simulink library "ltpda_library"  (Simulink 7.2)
settings: Solver=ode45  SolverMode=SingleTasking  StartTime=0.0  StopTime=10.0  RelTol=1e-3
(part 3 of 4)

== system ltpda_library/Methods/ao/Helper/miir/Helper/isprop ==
  In1 : Inport  OutDataType=sfix(16)  OutScaling=2^0
  isprop : M-S-Function  Tag=isprop  FunctionName=ltpdasim
  Out1 : Outport  OutDataType=sfix(16)  OutScaling=2^0
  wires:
  In1/1 -> isprop/1
  isprop/1 -> Out1/1

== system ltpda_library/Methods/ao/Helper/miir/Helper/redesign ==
  In1 : Inport  OutDataType=sfix(16)  OutScaling=2^0
  redesign : M-S-Function  Tag=redesign  FunctionName=ltpdasim
  Out1 : Outport  OutDataType=sfix(16)  OutScaling=2^0
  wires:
  In1/1 -> redesign/1
  redesign/1 -> Out1/1

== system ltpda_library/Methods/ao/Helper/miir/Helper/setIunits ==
  In1 : Inport  OutDataType=sfix(16)  OutScaling=2^0
  setIunits : M-S-Function  Tag=setIunits  FunctionName=ltpdasim
  Out1 : Outport  OutDataType=sfix(16)  OutScaling=2^0
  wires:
  In1/1 -> setIunits/1
  setIunits/1 -> Out1/1

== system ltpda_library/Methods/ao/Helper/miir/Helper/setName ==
  In1 : Inport  OutDataType=sfix(16)  OutScaling=2^0
  setName : M-S-Function  Tag=setName  FunctionName=ltpdasim
  Out1 : Outport  OutDataType=sfix(16)  OutScaling=2^0
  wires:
  In1/1 -> setName/1
  setName/1 -> Out1/1

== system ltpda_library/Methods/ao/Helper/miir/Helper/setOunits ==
  In1 : Inport  OutDataType=sfix(16)  OutScaling=2^0
  setOunits : M-S-Function  Tag=setOunits  FunctionName=ltpdasim
  Out1 : Outport  OutDataType=sfix(16)  OutScaling=2^0
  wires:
  In1/1 -> setOunits/1
  setOunits/1 -> Out1/1

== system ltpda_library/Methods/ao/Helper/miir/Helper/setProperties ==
  In1 : Inport  OutDataType=sfix(16)  OutScaling=2^0
  setProperties : M-S-Function  Tag=setProperties  FunctionName=ltpdasim
  Out1 : Outport  OutDataType=sfix(16)  OutScaling=2^0
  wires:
  In1/1 -> setProperties/1
  setProperties/1 -> Out1/1

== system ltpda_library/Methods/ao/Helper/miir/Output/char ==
  In1 : Inport  OutDataType=sfix(16)  OutScaling=2^0
  Terminator : Terminator
  char : M-S-Function  Tag=char  FunctionName=ltpdasim
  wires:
  char/1 -> Terminator/1
  In1/1 -> char/1

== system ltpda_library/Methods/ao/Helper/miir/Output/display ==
  In1 : Inport  OutDataType=sfix(16)  OutScaling=2^0
  Terminator : Terminator
  display : M-S-Function  Tag=display  FunctionName=ltpdasim
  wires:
  display/1 -> Terminator/1
  In1/1 -> display/1

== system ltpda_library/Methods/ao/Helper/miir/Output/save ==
  In1 : Inport  OutDataType=sfix(16)  OutScaling=2^0
  Terminator : Terminator
  report : M-S-Function  Tag=report  FunctionName=ltpdasim
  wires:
  report/1 -> Terminator/1
  In1/1 -> report/1

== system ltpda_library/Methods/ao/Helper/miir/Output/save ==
  In1 : Inport  OutDataType=sfix(16)  OutScaling=2^0
  Terminator : Terminator
  save : M-S-Function  Tag=save  FunctionName=ltpdasim
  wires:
  save/1 -> Terminator/1
  In1/1 -> save/1

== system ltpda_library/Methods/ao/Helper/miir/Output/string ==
  In1 : Inport  OutDataType=sfix(16)  OutScaling=2^0
  Terminator : Terminator
  string : M-S-Function  Tag=string  FunctionName=ltpdasim
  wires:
  string/1 -> Terminator/1
  In1/1 -> string/1

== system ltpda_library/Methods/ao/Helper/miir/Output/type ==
  In1 : Inport  OutDataType=sfix(16)  OutScaling=2^0
  Terminator : Terminator
  type : M-S-Function  Tag=type  FunctionName=ltpdasim
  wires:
  type/1 -> Terminator/1
  In1/1 -> type/1

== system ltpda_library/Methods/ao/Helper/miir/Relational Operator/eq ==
  In1 : Inport  OutDataType=sfix(16)  OutScaling=2^0
  eq : M-S-Function  Tag=eq  FunctionName=ltpdasim
  Out1 : Outport  OutDataType=sfix(16)  OutScaling=2^0
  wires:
  In1/1 -> eq/1
  eq/1 -> Out1/1

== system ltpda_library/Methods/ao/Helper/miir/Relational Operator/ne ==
  In1 : Inport  OutDataType=sfix(16)  OutScaling=2^0
  ne : M-S-Function  Tag=ne  FunctionName=ltpdasim
  Out1 : Outport  OutDataType=sfix(16)  OutScaling=2^0
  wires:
  In1/1 -> ne/1
  ne/1 -> Out1/1

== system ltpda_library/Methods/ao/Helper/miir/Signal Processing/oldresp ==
  In1 : Inport  OutDataType=sfix(16)  OutScaling=2^0
  oldresp : M-S-Function  Tag=oldresp  FunctionName=ltpdasim
  Out1 : Outport  OutDataType=sfix(16)  OutScaling=2^0
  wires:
  In1/1 -> oldresp/1
  oldresp/1 -> Out1/1

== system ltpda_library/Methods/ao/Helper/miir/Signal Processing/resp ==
  In1 : Inport  OutDataType=sfix(16)  OutScaling=2^0
  resp : M-S-Function  Tag=resp  FunctionName=ltpdasim
  Out1 : Outport  OutDataType=sfix(16)  OutScaling=2^0
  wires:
  In1/1 -> resp/1
  resp/1 -> Out1/1

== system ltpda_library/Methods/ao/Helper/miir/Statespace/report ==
  In1 : Inport  OutDataType=sfix(16)  OutScaling=2^0
  report : M-S-Function  Tag=report  FunctionName=ltpdasim
  Out1 : Outport  OutDataType=sfix(16)  OutScaling=2^0
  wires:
  In1/1 -> report/1
  report/1 -> Out1/1

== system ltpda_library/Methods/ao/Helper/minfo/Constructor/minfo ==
  Ground : Ground
  minfo : M-S-Function  Tag=minfo  FunctionName=ltpdasim
  Out1 : Outport  OutDataType=sfix(16)  OutScaling=2^0
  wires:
  Ground/1 -> minfo/1
  minfo/1 -> Out1/1

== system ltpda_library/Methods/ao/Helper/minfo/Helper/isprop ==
  In1 : Inport  OutDataType=sfix(16)  OutScaling=2^0
  isprop : M-S-Function  Tag=isprop  FunctionName=ltpdasim
  Out1 : Outport  OutDataType=sfix(16)  OutScaling=2^0
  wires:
  In1/1 -> isprop/1
  isprop/1 -> Out1/1

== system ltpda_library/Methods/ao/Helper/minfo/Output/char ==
  In1 : Inport  OutDataType=sfix(16)  OutScaling=2^0
  Terminator : Terminator
  char : M-S-Function  Tag=char  FunctionName=ltpdasim
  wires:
  char/1 -> Terminator/1
  In1/1 -> char/1

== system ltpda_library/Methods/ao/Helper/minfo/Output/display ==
  In1 : Inport  OutDataType=sfix(16)  OutScaling=2^0
  Terminator : Terminator
  display : M-S-Function  Tag=display  FunctionName=ltpdasim
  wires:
  display/1 -> Terminator/1
  In1/1 -> display/1

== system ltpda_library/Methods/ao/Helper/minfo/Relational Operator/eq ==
  In1 : Inport  OutDataType=sfix(16)  OutScaling=2^0
  eq : M-S-Function  Tag=eq  FunctionName=ltpdasim
  Out1 : Outport  OutDataType=sfix(16)  OutScaling=2^0
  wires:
  In1/1 -> eq/1
  eq/1 -> Out1/1

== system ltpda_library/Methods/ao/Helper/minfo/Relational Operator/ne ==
  In1 : Inport  OutDataType=sfix(16)  OutScaling=2^0
  ne : M-S-Function  Tag=ne  FunctionName=ltpdasim
  Out1 : Outport  OutDataType=sfix(16)  OutScaling=2^0
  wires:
  In1/1 -> ne/1
  ne/1 -> Out1/1

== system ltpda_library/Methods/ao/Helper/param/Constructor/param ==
  Ground : Ground
  param : M-S-Function  Tag=param  FunctionName=ltpdasim
  Out1 : Outport  OutDataType=sfix(16)  OutScaling=2^0
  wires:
  Ground/1 -> param/1
  param/1 -> Out1/1

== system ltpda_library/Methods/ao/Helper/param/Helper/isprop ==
  In1 : Inport  OutDataType=sfix(16)  OutScaling=2^0
  isprop : M-S-Function  Tag=isprop  FunctionName=ltpdasim
  Out1 : Outport  OutDataType=sfix(16)  OutScaling=2^0
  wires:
  In1/1 -> isprop/1
  isprop/1 -> Out1/1

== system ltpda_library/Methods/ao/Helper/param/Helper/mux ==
  In1 : Inport  OutDataType=sfix(16)  OutScaling=2^0
  mux : M-S-Function  Tag=mux  FunctionName=ltpdasim
  Out1 : Outport  OutDataType=sfix(16)  OutScaling=2^0
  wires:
  In1/1 -> mux/1
  mux/1 -> Out1/1

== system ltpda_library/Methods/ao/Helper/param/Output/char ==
  In1 : Inport  OutDataType=sfix(16)  OutScaling=2^0
  Terminator : Terminator
  char : M-S-Function  Tag=char  FunctionName=ltpdasim
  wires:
  char/1 -> Terminator/1
  In1/1 -> char/1

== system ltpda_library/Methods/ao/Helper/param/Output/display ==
  In1 : Inport  OutDataType=sfix(16)  OutScaling=2^0
  Terminator : Terminator
  display : M-S-Function  Tag=display  FunctionName=ltpdasim
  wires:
  display/1 -> Terminator/1
  In1/1 -> display/1

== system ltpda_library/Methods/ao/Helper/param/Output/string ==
  In1 : Inport  OutDataType=sfix(16)  OutScaling=2^0
  Terminator : Terminator
  string : M-S-Function  Tag=string  FunctionName=ltpdasim
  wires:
  string/1 -> Terminator/1
  In1/1 -> string/1

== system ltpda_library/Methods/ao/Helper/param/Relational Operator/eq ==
  In1 : Inport  OutDataType=sfix(16)  OutScaling=2^0
  eq : M-S-Function  Tag=eq  FunctionName=ltpdasim
  Out1 : Outport  OutDataType=sfix(16)  OutScaling=2^0
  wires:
  In1/1 -> eq/1
  eq/1 -> Out1/1

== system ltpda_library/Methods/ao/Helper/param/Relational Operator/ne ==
  In1 : Inport  OutDataType=sfix(16)  OutScaling=2^0
  ne : M-S-Function  Tag=ne  FunctionName=ltpdasim
  Out1 : Outport  OutDataType=sfix(16)  OutScaling=2^0
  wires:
  In1/1 -> ne/1
  ne/1 -> Out1/1

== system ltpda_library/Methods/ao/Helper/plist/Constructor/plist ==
  Ground : Ground
  plist : M-S-Function  Tag=plist  FunctionName=ltpdasim
  Out1 : Outport  OutDataType=sfix(16)  OutScaling=2^0
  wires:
  Ground/1 -> plist/1
  ?parfrac/1 -> Out1/1

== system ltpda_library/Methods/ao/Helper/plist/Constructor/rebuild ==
  Ground : Ground
  rebuild : M-S-Function  Tag=rebuild  FunctionName=ltpdasim
  Out1 : Outport  OutDataType=sfix(16)  OutScaling=2^0
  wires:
  Ground/1 -> rebuild/1
  rebuild/1 -> Out1/1

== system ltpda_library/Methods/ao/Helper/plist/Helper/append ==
  In1 : Inport  OutDataType=sfix(16)  OutScaling=2^0
  append : M-S-Function  Tag=append  FunctionName=ltpdasim
  Out1 : Outport  OutDataType=sfix(16)  OutScaling=2^0
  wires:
  In1/1 -> append/1
  append/1 -> Out1/1

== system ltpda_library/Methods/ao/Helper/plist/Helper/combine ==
  In1 : Inport  OutDataType=sfix(16)  OutScaling=2^0
  combine : M-S-Function  Tag=combine  FunctionName=ltpdasim
  Out1 : Outport  OutDataType=sfix(16)  OutScaling=2^0
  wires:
  In1/1 -> combine/1
  combine/1 -> Out1/1

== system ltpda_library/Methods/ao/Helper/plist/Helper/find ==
  In1 : Inport  OutDataType=sfix(16)  OutScaling=2^0
  find : M-S-Function  Tag=find  FunctionName=ltpdasim
  Out1 : Outport  OutDataType=sfix(16)  OutScaling=2^0
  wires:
  In1/1 -> find/1
  find/1 -> Out1/1

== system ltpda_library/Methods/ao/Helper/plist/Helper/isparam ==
  In1 : Inport  OutDataType=sfix(16)  OutScaling=2^0
  isparam : M-S-Function  Tag=isparam  FunctionName=ltpdasim
  Out1 : Outport  OutDataType=sfix(16)  OutScaling=2^0
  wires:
  In1/1 -> isparam/1
  isparam/1 -> Out1/1

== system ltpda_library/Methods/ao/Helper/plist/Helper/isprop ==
  In1 : Inport  OutDataType=sfix(16)  OutScaling=2^0
  isprop : M-S-Function  Tag=isprop  FunctionName=ltpdasim
  Out1 : Outport  OutDataType=sfix(16)  OutScaling=2^0
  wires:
  In1/1 -> isprop/1
  isprop/1 -> Out1/1

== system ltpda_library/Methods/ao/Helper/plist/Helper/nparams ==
  In1 : Inport  OutDataType=sfix(16)  OutScaling=2^0
  nparams : M-S-Function  Tag=nparams  FunctionName=ltpdasim
  Out1 : Outport  OutDataType=sfix(16)  OutScaling=2^0
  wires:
  In1/1 -> nparams/1
  nparams/1 -> Out1/1

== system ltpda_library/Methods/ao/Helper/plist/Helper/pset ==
  In1 : Inport  OutDataType=sfix(16)  OutScaling=2^0
  pset : M-S-Function  Tag=pset  FunctionName=ltpdasim
  Out1 : Outport  OutDataType=sfix(16)  OutScaling=2^0
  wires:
  In1/1 -> pset/1
  pset/1 -> Out1/1

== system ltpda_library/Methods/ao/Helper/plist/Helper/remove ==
  In1 : Inport  OutDataType=sfix(16)  OutScaling=2^0
  remove : M-S-Function  Tag=remove  FunctionName=ltpdasim
  Out1 : Outport  OutDataType=sfix(16)  OutScaling=2^0
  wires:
  In1/1 -> remove/1
  remove/1 -> Out1/1

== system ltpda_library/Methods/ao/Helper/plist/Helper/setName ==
  In1 : Inport  OutDataType=sfix(16)  OutScaling=2^0
  setName : M-S-Function  Tag=setName  FunctionName=ltpdasim
  Out1 : Outport  OutDataType=sfix(16)  OutScaling=2^0
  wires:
  In1/1 -> setName/1
  setName/1 -> Out1/1

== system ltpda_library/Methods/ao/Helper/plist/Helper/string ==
  In1 : Inport  OutDataType=sfix(16)  OutScaling=2^0
  string : M-S-Function  Tag=string  FunctionName=ltpdasim
  Out1 : Outport  OutDataType=sfix(16)  OutScaling=2^0
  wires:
  In1/1 -> string/1
  string/1 -> Out1/1

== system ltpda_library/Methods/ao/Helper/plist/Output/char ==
  In1 : Inport  OutDataType=sfix(16)  OutScaling=2^0
  Terminator : Terminator
  char : M-S-Function  Tag=char  FunctionName=ltpdasim
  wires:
  char/1 -> Terminator/1
  In1/1 -> char/1

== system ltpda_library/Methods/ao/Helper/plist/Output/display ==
  In1 : Inport  OutDataType=sfix(16)  OutScaling=2^0
  Terminator : Terminator
  display : M-S-Function  Tag=display  FunctionName=ltpdasim
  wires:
  display/1 -> Terminator/1
  In1/1 -> display/1

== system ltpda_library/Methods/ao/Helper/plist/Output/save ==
  In1 : Inport  OutDataType=sfix(16)  OutScaling=2^0
  Terminator : Terminator
  save : M-S-Function  Tag=save  FunctionName=ltpdasim
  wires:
  save/1 -> Terminator/1
  In1/1 -> save/1

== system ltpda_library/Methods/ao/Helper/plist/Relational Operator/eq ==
  In1 : Inport  OutDataType=sfix(16)  OutScaling=2^0
  eq : M-S-Function  Tag=eq  FunctionName=ltpdasim
  Out1 : Outport  OutDataType=sfix(16)  OutScaling=2^0
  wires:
  In1/1 -> eq/1
  eq/1 -> Out1/1

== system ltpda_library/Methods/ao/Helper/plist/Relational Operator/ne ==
  In1 : Inport  OutDataType=sfix(16)  OutScaling=2^0
  ne : M-S-Function  Tag=ne  FunctionName=ltpdasim
  Out1 : Outport  OutDataType=sfix(16)  OutScaling=2^0
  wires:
  In1/1 -> ne/1
  ne/1 -> Out1/1

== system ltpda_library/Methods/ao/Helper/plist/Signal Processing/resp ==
  In1 : Inport  OutDataType=sfix(16)  OutScaling=2^0
  resp : M-S-Function  Tag=resp  FunctionName=ltpdasim
  Out1 : Outport  OutDataType=sfix(16)  OutScaling=2^0
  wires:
  In1/1 -> resp/1
  resp/1 -> Out1/1

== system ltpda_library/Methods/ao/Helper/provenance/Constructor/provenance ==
  Ground : Ground
  provenance : M-S-Function  Tag=provenance  FunctionName=ltpdasim
  Out1 : Outport  OutDataType=sfix(16)  OutScaling=2^0
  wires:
  Ground/1 -> provenance/1
  provenance/1 -> Out1/1

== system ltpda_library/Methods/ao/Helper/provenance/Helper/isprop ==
  In1 : Inport  OutDataType=sfix(16)  OutScaling=2^0
  isprop : M-S-Function  Tag=isprop  FunctionName=ltpdasim
  Out1 : Outport  OutDataType=sfix(16)  OutScaling=2^0
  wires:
  In1/1 -> isprop/1
  isprop/1 -> Out1/1

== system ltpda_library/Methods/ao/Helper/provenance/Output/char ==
  In1 : Inport  OutDataType=sfix(16)  OutScaling=2^0
  Terminator : Terminator
  char : M-S-Function  Tag=char  FunctionName=ltpdasim
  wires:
  char/1 -> Terminator/1
  In1/1 -> char/1

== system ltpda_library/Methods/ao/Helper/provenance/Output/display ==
  In1 : Inport  OutDataType=sfix(16)  OutScaling=2^0
  Terminator : Terminator
  display : M-S-Function  Tag=display  FunctionName=ltpdasim
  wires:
  display/1 -> Terminator/1
  In1/1 -> display/1

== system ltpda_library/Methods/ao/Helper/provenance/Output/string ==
  In1 : Inport  OutDataType=sfix(16)  OutScaling=2^0
  Terminator : Terminator
  string : M-S-Function  Tag=string  FunctionName=ltpdasim
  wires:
  string/1 -> Terminator/1
  In1/1 -> string/1

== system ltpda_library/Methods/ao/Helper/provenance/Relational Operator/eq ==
  In1 : Inport  OutDataType=sfix(16)  OutScaling=2^0
  eq : M-S-Function  Tag=eq  FunctionName=ltpdasim
  Out1 : Outport  OutDataType=sfix(16)  OutScaling=2^0
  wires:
  In1/1 -> eq/1
  eq/1 -> Out1/1

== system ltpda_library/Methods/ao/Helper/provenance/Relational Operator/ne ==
  In1 : Inport  OutDataType=sfix(16)  OutScaling=2^0
  ne : M-S-Function  Tag=ne  FunctionName=ltpdasim
  Out1 : Outport  OutDataType=sfix(16)  OutScaling=2^0
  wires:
  In1/1 -> ne/1
  ne/1 -> Out1/1

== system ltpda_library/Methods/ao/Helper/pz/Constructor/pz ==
  Ground : Ground
  pz : M-S-Function  Tag=pz  FunctionName=ltpdasim
  Out1 : Outport  OutDataType=sfix(16)  OutScaling=2^0
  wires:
  Ground/1 -> pz/1
  pz/1 -> Out1/1

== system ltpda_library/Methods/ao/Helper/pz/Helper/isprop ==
  In1 : Inport  OutDataType=sfix(16)  OutScaling=2^0
  isprop : M-S-Function  Tag=isprop  FunctionName=ltpdasim
  Out1 : Outport  OutDataType=sfix(16)  OutScaling=2^0
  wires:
  In1/1 -> isprop/1
  isprop/1 -> Out1/1

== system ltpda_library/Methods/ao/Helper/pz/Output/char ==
  In1 : Inport  OutDataType=sfix(16)  OutScaling=2^0
  Terminator : Terminator
  char : M-S-Function  Tag=char  FunctionName=ltpdasim
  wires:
  char/1 -> Terminator/1
  In1/1 -> char/1

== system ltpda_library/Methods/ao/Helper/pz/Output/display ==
  In1 : Inport  OutDataType=sfix(16)  OutScaling=2^0
  Terminator : Terminator
  display : M-S-Function  Tag=display  FunctionName=ltpdasim
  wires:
  display/1 -> Terminator/1
  In1/1 -> display/1

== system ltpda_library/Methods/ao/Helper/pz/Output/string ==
  In1 : Inport  OutDataType=sfix(16)  OutScaling=2^0
  Terminator : Terminator
  string : M-S-Function  Tag=string  FunctionName=ltpdasim
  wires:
  string/1 -> Terminator/1
  In1/1 -> string/1

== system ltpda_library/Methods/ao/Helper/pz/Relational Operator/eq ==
  In1 : Inport  OutDataType=sfix(16)  OutScaling=2^0
  eq : M-S-Function  Tag=eq  FunctionName=ltpdasim
  Out1 : Outport  OutDataType=sfix(16)  OutScaling=2^0
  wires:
  In1/1 -> eq/1
  eq/1 -> Out1/1

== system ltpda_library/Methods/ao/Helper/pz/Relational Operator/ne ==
  In1 : Inport  OutDataType=sfix(16)  OutScaling=2^0
  ne : M-S-Function  Tag=ne  FunctionName=ltpdasim
  Out1 : Outport  OutDataType=sfix(16)  OutScaling=2^0
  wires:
  In1/1 -> ne/1
  ne/1 -> Out1/1

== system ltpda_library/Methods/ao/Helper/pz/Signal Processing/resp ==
  In1 : Inport  OutDataType=sfix(16)  OutScaling=2^0
  resp : M-S-Function  Tag=resp  FunctionName=ltpdasim
  Out1 : Outport  OutDataType=sfix(16)  OutScaling=2^0
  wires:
  In1/1 -> resp/1
  resp/1 -> Out1/1

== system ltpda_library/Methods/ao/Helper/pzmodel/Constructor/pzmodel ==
  Ground : Ground
  pzmodel : M-S-Function  Tag=pzmodel  FunctionName=ltpdasim
  Out1 : Outport  OutDataType=sfix(16)  OutScaling=2^0
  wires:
  Ground/1 -> pzmodel/1
  pzmodel/1 -> Out1/1

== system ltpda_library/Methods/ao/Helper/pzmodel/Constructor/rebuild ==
  Ground : Ground
  rebuild : M-S-Function  Tag=rebuild  FunctionName=ltpdasim
  Out1 : Outport  OutDataType=sfix(16)  OutScaling=2^0
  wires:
  Ground/1 -> rebuild/1
  rebuild/1 -> Out1/1

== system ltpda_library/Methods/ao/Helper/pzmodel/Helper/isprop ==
  In1 : Inport  OutDataType=sfix(16)  OutScaling=2^0
  isprop : M-S-Function  Tag=isprop  FunctionName=ltpdasim
  Out1 : Outport  OutDataType=sfix(16)  OutScaling=2^0
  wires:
  In1/1 -> isprop/1
  isprop/1 -> Out1/1

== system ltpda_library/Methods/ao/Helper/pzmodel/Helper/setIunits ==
  In1 : Inport  OutDataType=sfix(16)  OutScaling=2^0
  setIunits : M-S-Function  Tag=setIunits  FunctionName=ltpdasim
  Out1 : Outport  OutDataType=sfix(16)  OutScaling=2^0
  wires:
  In1/1 -> setIunits/1
  setIunits/1 -> Out1/1

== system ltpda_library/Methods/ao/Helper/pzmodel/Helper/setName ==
  In1 : Inport  OutDataType=sfix(16)  OutScaling=2^0
  setName : M-S-Function  Tag=setName  FunctionName=ltpdasim
  Out1 : Outport  OutDataType=sfix(16)  OutScaling=2^0
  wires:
  In1/1 -> setName/1
  setName/1 -> Out1/1

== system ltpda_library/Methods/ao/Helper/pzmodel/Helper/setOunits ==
  In1 : Inport  OutDataType=sfix(16)  OutScaling=2^0
  setOunits : M-S-Function  Tag=setOunits  FunctionName=ltpdasim
  Out1 : Outport  OutDataType=sfix(16)  OutScaling=2^0
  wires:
  In1/1 -> setOunits/1
  setOunits/1 -> Out1/1

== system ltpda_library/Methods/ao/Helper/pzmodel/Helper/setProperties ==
  In1 : Inport  OutDataType=sfix(16)  OutScaling=2^0
  setProperties : M-S-Function  Tag=setProperties  FunctionName=ltpdasim
  Out1 : Outport  OutDataType=sfix(16)  OutScaling=2^0
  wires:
  In1/1 -> setProperties/1
  setProperties/1 -> Out1/1

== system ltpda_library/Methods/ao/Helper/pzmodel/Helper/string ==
  In1 : Inport  OutDataType=sfix(16)  OutScaling=2^0
  string : M-S-Function  Tag=string  FunctionName=ltpdasim
  Out1 : Outport  OutDataType=sfix(16)  OutScaling=2^0
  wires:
  In1/1 -> string/1
  string/1 -> Out1/1

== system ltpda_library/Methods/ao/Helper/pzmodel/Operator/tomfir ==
  In1 : Inport  OutDataType=sfix(16)  OutScaling=2^0
  tomfir : M-S-Function  Tag=tomfir  FunctionName=ltpdasim
  Out1 : Outport  OutDataType=sfix(16)  OutScaling=2^0
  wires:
  In1/1 -> tomfir/1
  tomfir/1 -> Out1/1

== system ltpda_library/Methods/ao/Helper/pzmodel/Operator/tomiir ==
  In1 : Inport  OutDataType=sfix(16)  OutScaling=2^0
  tomiir : M-S-Function  Tag=tomiir  FunctionName=ltpdasim
  Out1 : Outport  OutDataType=sfix(16)  OutScaling=2^0
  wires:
  In1/1 -> tomiir/1
  tomiir/1 -> Out1/1

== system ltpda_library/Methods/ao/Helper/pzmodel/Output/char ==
  In1 : Inport  OutDataType=sfix(16)  OutScaling=2^0
  Terminator : Terminator
  char : M-S-Function  Tag=char  FunctionName=ltpdasim
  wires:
  char/1 -> Terminator/1
  In1/1 -> char/1

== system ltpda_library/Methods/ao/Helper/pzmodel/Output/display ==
  In1 : Inport  OutDataType=sfix(16)  OutScaling=2^0
  Terminator : Terminator
  display : M-S-Function  Tag=display  FunctionName=ltpdasim
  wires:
  display/1 -> Terminator/1
  In1/1 -> display/1

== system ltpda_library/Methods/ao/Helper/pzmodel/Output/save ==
  In1 : Inport  OutDataType=sfix(16)  OutScaling=2^0
  Terminator : Terminator
  save : M-S-Function  Tag=save  FunctionName=ltpdasim
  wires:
  save/1 -> Terminator/1
  In1/1 -> save/1

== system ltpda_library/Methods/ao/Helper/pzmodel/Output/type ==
  In1 : Inport  OutDataType=sfix(16)  OutScaling=2^0
  Terminator : Terminator
  type : M-S-Function  Tag=type  FunctionName=ltpdasim
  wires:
  type/1 -> Terminator/1
  In1/1 -> type/1

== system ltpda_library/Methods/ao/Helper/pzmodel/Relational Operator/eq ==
  In1 : Inport  OutDataType=sfix(16)  OutScaling=2^0
  eq : M-S-Function  Tag=eq  FunctionName=ltpdasim
  Out1 : Outport  OutDataType=sfix(16)  OutScaling=2^0
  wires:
  In1/1 -> eq/1
  eq/1 -> Out1/1

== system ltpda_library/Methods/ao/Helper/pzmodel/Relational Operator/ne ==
  In1 : Inport  OutDataType=sfix(16)  OutScaling=2^0
  ne : M-S-Function  Tag=ne  FunctionName=ltpdasim
  Out1 : Outport  OutDataType=sfix(16)  OutScaling=2^0
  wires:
  In1/1 -> ne/1
  ne/1 -> Out1/1

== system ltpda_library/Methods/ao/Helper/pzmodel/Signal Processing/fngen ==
  In1 : Inport  OutDataType=sfix(16)  OutScaling=2^0
  fngen : M-S-Function  Tag=fngen  FunctionName=ltpdasim
  Out1 : Outport  OutDataType=sfix(16)  OutScaling=2^0
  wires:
  In1/1 -> fngen/1
  fngen/1 -> Out1/1

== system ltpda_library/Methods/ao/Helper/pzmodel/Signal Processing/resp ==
  In1 : Inport  OutDataType=sfix(16)  OutScaling=2^0
  resp : M-S-Function  Tag=resp  FunctionName=ltpdasim
  Out1 : Outport  OutDataType=sfix(16)  OutScaling=2^0
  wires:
  In1/1 -> resp/1
  resp/1 -> Out1/1

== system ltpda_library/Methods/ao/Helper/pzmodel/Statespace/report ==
  In1 : Inport  OutDataType=sfix(16)  OutScaling=2^0
  report : M-S-Function  Tag=report  FunctionName=ltpdasim
  Out1 : Outport  OutDataType=sfix(16)  OutScaling=2^0
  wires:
  In1/1 -> report/1
  ?lisovfit/1 -> Out1/1

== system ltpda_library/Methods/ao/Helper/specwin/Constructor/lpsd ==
  In1 : Inport  OutDataType=sfix(16)  OutScaling=2^0
  lpsd : M-S-Function  Tag=lpsd  FunctionName=ltpdasim
  Out1 : Outport  OutDataType=sfix(16)  OutScaling=2^0
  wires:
  In1/1 -> lpsd/1
  lpsd/1 -> Out1/1

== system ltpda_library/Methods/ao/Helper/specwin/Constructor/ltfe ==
  In1 : Inport  OutDataType=sfix(16)  OutScaling=2^0
  ltfe : M-S-Function  Tag=ltfe  FunctionName=ltpdasim
  Out1 : Outport  OutDataType=sfix(16)  OutScaling=2^0
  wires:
  In1/1 -> ltfe/1
  ltfe/1 -> Out1/1

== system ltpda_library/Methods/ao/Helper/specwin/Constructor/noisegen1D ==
  In1 : Inport  OutDataType=sfix(16)  OutScaling=2^0
  noisegen1D : M-S-Function  Tag=noisegen1D  FunctionName=ltpdasim
  Out1 : Outport  OutDataType=sfix(16)  OutScaling=2^0
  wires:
  In1/1 -> noisegen1D/1
  noisegen1D/1 -> Out1/1

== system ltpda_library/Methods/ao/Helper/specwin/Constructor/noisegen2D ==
  In1 : Inport  OutDataType=sfix(16)  OutScaling=2^0
  noisegen2D : M-S-Function  Tag=noisegen2D  FunctionName=ltpdasim
  Out1 : Outport  OutDataType=sfix(16)  OutScaling=2^0
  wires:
  In1/1 -> noisegen2D/1
  noisegen2D/1 -> Out1/1

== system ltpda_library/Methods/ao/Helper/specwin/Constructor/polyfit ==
  In1 : Inport  OutDataType=sfix(16)  OutScaling=2^0
  polyfit : M-S-Function  Tag=polyfit  FunctionName=ltpdasim
  Out1 : Outport  OutDataType=sfix(16)  OutScaling=2^0
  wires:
  In1/1 -> polyfit/1
  polyfit/1 -> Out1/1

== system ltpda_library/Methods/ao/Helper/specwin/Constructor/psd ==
  In1 : Inport  OutDataType=sfix(16)  OutScaling=2^0
  psd : M-S-Function  Tag=psd  FunctionName=ltpdasim
  Out1 : Outport  OutDataType=sfix(16)  OutScaling=2^0
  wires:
  In1/1 -> psd/1
  psd/1 -> Out1/1

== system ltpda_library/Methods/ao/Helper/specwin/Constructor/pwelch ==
  In1 : Inport  OutDataType=sfix(16)  OutScaling=2^0
  pwelch : M-S-Function  Tag=pwelch  FunctionName=ltpdasim
  Out1 : Outport  OutDataType=sfix(16)  OutScaling=2^0
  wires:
  In1/1 -> pwelch/1
  pwelch/1 -> Out1/1

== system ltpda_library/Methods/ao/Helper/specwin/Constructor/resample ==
  In1 : Inport  OutDataType=sfix(16)  OutScaling=2^0
  resample : M-S-Function  Tag=resample  FunctionName=ltpdasim
  Out1 : Outport  OutDataType=sfix(16)  OutScaling=2^0
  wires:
  In1/1 -> resample/1
  resample/1 -> Out1/1

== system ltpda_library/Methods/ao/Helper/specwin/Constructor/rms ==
  In1 : Inport  OutDataType=sfix(16)  OutScaling=2^0
  rms : M-S-Function  Tag=rms  FunctionName=ltpdasim
  Out1 : Outport  OutDataType=sfix(16)  OutScaling=2^0
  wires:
  In1/1 -> rms/1
  rms/1 -> Out1/1

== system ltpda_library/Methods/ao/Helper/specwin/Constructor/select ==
  In1 : Inport  OutDataType=sfix(16)  OutScaling=2^0
  select : M-S-Function  Tag=select  FunctionName=ltpdasim
  Out1 : Outport  OutDataType=sfix(16)  OutScaling=2^0
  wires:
  In1/1 -> select/1
  select/1 -> Out1/1

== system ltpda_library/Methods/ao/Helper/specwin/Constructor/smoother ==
  In1 : Inport  OutDataType=sfix(16)  OutScaling=2^0
  smoother : M-S-Function  Tag=smoother  FunctionName=ltpdasim
  Out1 : Outport  OutDataType=sfix(16)  OutScaling=2^0
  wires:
  In1/1 -> smoother/1
  smoother/1 -> Out1/1

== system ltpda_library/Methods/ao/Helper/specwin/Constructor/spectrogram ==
  In1 : Inport  OutDataType=sfix(16)  OutScaling=2^0
  spectrogram : M-S-Function  Tag=spectrogram  FunctionName=ltpdasim
  Out1 : Outport  OutDataType=sfix(16)  OutScaling=2^0
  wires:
  In1/1 -> spectrogram/1
  spectrogram/1 -> Out1/1

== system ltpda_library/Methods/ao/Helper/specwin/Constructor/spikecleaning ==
  In1 : Inport  OutDataType=sfix(16)  OutScaling=2^0
  spikecleaning : M-S-Function  Tag=spikecleaning  FunctionName=ltpdasim
  Out1 : Outport  OutDataType=sfix(16)  OutScaling=2^0
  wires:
  In1/1 -> spikecleaning/1
  spikecleaning/1 -> Out1/1

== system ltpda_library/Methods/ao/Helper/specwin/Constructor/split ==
  In1 : Inport  OutDataType=sfix(16)  OutScaling=2^0
  split : M-S-Function  Tag=split  FunctionName=ltpdasim
  Out1 : Outport  OutDataType=sfix(16)  OutScaling=2^0
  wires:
  In1/1 -> split/1
  split/1 -> Out1/1

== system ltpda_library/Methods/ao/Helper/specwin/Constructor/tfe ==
  In1 : Inport  OutDataType=sfix(16)  OutScaling=2^0
  tfe : M-S-Function  Tag=tfe  FunctionName=ltpdasim
  Out1 : Outport  OutDataType=sfix(16)  OutScaling=2^0
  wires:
  In1/1 -> tfe/1
  tfe/1 -> Out1/1

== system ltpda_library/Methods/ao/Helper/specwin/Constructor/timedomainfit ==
  In1 : Inport  OutDataType=sfix(16)  OutScaling=2^0
  timedomainfit : M-S-Function  Tag=timedomainfit  FunctionName=ltpdasim
  Out1 : Outport  OutDataType=sfix(16)  OutScaling=2^0
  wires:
  In1/1 -> timedomainfit/1
  timedomainfit/1 -> Out1/1

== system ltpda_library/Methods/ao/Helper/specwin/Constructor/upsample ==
  In1 : Inport  OutDataType=sfix(16)  OutScaling=2^0
  upsample : M-S-Function  Tag=upsample  FunctionName=ltpdasim
  Out1 : Outport  OutDataType=sfix(16)  OutScaling=2^0
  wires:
  In1/1 -> upsample/1
  upsample/1 -> Out1/1

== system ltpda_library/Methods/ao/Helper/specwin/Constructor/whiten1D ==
  In1 : Inport  OutDataType=sfix(16)  OutScaling=2^0
  whiten1D : M-S-Function  Tag=whiten1D  FunctionName=ltpdasim
  Out1 : Outport  OutDataType=sfix(16)  OutScaling=2^0
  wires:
  In1/1 -> whiten1D/1
  whiten1D/1 -> Out1/1

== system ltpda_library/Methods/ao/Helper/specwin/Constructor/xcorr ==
  In1 : Inport  OutDataType=sfix(16)  OutScaling=2^0
  xcorr : M-S-Function  Tag=xcorr  FunctionName=ltpdasim
  Out1 : Outport  OutDataType=sfix(16)  OutScaling=2^0
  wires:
  In1/1 -> xcorr/1
  xcorr/1 -> Out1/1

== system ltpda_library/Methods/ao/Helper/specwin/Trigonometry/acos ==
  In1 : Inport  OutDataType=sfix(16)  OutScaling=2^0
  acos : M-S-Function  Tag=acos  FunctionName=ltpdasim
  Out1 : Outport  OutDataType=sfix(16)  OutScaling=2^0
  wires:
  In1/1 -> acos/1
  acos/1 -> Out1/1

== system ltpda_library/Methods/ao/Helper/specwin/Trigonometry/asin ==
  In1 : Inport  OutDataType=sfix(16)  OutScaling=2^0
  asin : M-S-Function  Tag=asin  FunctionName=ltpdasim
  Out1 : Outport  OutDataType=sfix(16)  OutScaling=2^0
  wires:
  In1/1 -> asin/1
  asin/1 -> Out1/1

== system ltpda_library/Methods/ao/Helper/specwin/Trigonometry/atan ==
  In1 : Inport  OutDataType=sfix(16)  OutScaling=2^0
  atan : M-S-Function  Tag=atan  FunctionName=ltpdasim
  Out1 : Outport  OutDataType=sfix(16)  OutScaling=2^0
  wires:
  In1/1 -> atan/1
  atan/1 -> Out1/1

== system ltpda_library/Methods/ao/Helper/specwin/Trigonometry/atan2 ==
  In1 : Inport  OutDataType=sfix(16)  OutScaling=2^0
  atan2 : M-S-Function  Tag=atan2  FunctionName=ltpdasim
  Out1 : Outport  OutDataType=sfix(16)  OutScaling=2^0
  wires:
  In1/1 -> atan2/1
  atan2/1 -> Out1/1

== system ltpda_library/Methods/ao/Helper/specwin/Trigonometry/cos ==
  In1 : Inport  OutDataType=sfix(16)  OutScaling=2^0
  cos : M-S-Function  Tag=cos  FunctionName=ltpdasim
  Out1 : Outport  OutDataType=sfix(16)  OutScaling=2^0
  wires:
  In1/1 -> cos/1
  cos/1 -> Out1/1

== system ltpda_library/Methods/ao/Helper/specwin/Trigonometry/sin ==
  In1 : Inport  OutDataType=sfix(16)  OutScaling=2^0
  sin : M-S-Function  Tag=sin  FunctionName=ltpdasim
  Out1 : Outport  OutDataType=sfix(16)  OutScaling=2^0
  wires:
  In1/1 -> sin/1
  sin/1 -> Out1/1

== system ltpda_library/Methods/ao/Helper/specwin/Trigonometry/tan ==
  In1 : Inport  OutDataType=sfix(16)  OutScaling=2^0
  tan : M-S-Function  Tag=tan  FunctionName=ltpdasim
  Out1 : Outport  OutDataType=sfix(16)  OutScaling=2^0
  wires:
  In1/1 -> tan/1
  tan/1 -> Out1/1

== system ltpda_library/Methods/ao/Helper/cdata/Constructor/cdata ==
  Ground : Ground
  cdata : M-S-Function  Tag=cdata  FunctionName=ltpdasim
  Out1 : Outport  OutDataType=sfix(16)  OutScaling=2^0
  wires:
  Ground/1 -> cdata/1
  cdata/1 -> Out1/1

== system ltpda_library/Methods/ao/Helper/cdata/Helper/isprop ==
  In1 : Inport  OutDataType=sfix(16)  OutScaling=2^0
  isprop : M-S-Function  Tag=isprop  FunctionName=ltpdasim
  Out1 : Outport  OutDataType=sfix(16)  OutScaling=2^0
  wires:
  In1/1 -> isprop/1
  isprop/1 -> Out1/1

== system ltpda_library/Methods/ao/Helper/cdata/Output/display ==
  In1 : Inport  OutDataType=sfix(16)  OutScaling=2^0
  Terminator : Terminator
  display : M-S-Function  Tag=display  FunctionName=ltpdasim
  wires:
  display/1 -> Terminator/1
  In1/1 -> display/1

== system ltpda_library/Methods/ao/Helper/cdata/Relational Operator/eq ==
  In1 : Inport  OutDataType=sfix(16)  OutScaling=2^0
  eq : M-S-Function  Tag=eq  FunctionName=ltpdasim
  Out1 : Outport  OutDataType=sfix(16)  OutScaling=2^0
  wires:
  In1/1 -> eq/1
  eq/1 -> Out1/1

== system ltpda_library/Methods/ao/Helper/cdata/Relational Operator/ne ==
  In1 : Inport  OutDataType=sfix(16)  OutScaling=2^0
  ne : M-S-Function  Tag=ne  FunctionName=ltpdasim
  Out1 : Outport  OutDataType=sfix(16)  OutScaling=2^0
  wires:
  In1/1 -> ne/1
  ne/1 -> Out1/1

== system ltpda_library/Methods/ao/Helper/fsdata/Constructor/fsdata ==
  Ground : Ground
  fsdata : M-S-Function  Tag=fsdata  FunctionName=ltpdasim
  Out1 : Outport  OutDataType=sfix(16)  OutScaling=2^0
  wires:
  Ground/1 -> fsdata/1
  fsdata/1 -> Out1/1

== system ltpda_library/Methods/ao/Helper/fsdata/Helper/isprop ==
  In1 : Inport  OutDataType=sfix(16)  OutScaling=2^0
  isprop : M-S-Function  Tag=isprop  FunctionName=ltpdasim
  Out1 : Outport  OutDataType=sfix(16)  OutScaling=2^0
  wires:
  In1/1 -> isprop/1
  isprop/1 -> Out1/1

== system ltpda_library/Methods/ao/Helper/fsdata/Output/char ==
  In1 : Inport  OutDataType=sfix(16)  OutScaling=2^0
  Terminator : Terminator
  char : M-S-Function  Tag=char  FunctionName=ltpdasim
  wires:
  char/1 -> Terminator/1
  In1/1 -> char/1

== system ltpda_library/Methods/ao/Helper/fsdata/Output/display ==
  In1 : Inport  OutDataType=sfix(16)  OutScaling=2^0
  Terminator : Terminator
  display : M-S-Function  Tag=display  FunctionName=ltpdasim
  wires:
  display/1 -> Terminator/1
  In1/1 -> display/1

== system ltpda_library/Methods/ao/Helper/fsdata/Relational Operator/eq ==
  In1 : Inport  OutDataType=sfix(16)  OutScaling=2^0
  eq : M-S-Function  Tag=eq  FunctionName=ltpdasim
  Out1 : Outport  OutDataType=sfix(16)  OutScaling=2^0
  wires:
  In1/1 -> eq/1
  eq/1 -> Out1/1

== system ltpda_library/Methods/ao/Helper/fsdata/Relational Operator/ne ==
  In1 : Inport  OutDataType=sfix(16)  OutScaling=2^0
  ne : M-S-Function  Tag=ne  FunctionName=ltpdasim
  Out1 : Outport  OutDataType=sfix(16)  OutScaling=2^0
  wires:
  In1/1 -> ne/1
  ne/1 -> Out1/1

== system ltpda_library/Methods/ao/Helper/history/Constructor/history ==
  Ground : Ground
  history : M-S-Function  Tag=history  FunctionName=ltpdasim
  Out1 : Outport  OutDataType=sfix(16)  OutScaling=2^0
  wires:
  Ground/1 -> history/1
  history/1 -> Out1/1

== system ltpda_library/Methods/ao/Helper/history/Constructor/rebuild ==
  Ground : Ground
  rebuild : M-S-Function  Tag=rebuild  FunctionName=ltpdasim
  Out1 : Outport  OutDataType=sfix(16)  OutScaling=2^0
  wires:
  Ground/1 -> rebuild/1
  rebuild/1 -> Out1/1

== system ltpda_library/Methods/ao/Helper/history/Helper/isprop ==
  In1 : Inport  OutDataType=sfix(16)  OutScaling=2^0
  isprop : M-S-Function  Tag=isprop  FunctionName=ltpdasim
  Out1 : Outport  OutDataType=sfix(16)  OutScaling=2^0
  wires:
  In1/1 -> isprop/1
  isprop/1 -> Out1/1

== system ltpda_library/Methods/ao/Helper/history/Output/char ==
  In1 : Inport  OutDataType=sfix(16)  OutScaling=2^0
  Terminator : Terminator
  char : M-S-Function  Tag=char  FunctionName=ltpdasim
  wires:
  char/1 -> Terminator/1
  In1/1 -> char/1

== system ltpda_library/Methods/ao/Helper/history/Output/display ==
  In1 : Inport  OutDataType=sfix(16)  OutScaling=2^0
  Terminator : Terminator
  display : M-S-Function  Tag=display  FunctionName=ltpdasim
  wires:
  display/1 -> Terminator/1
  In1/1 -> display/1

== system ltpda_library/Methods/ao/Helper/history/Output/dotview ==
  In1 : Inport  OutDataType=sfix(16)  OutScaling=2^0
  Terminator : Terminator
  dotview : M-S-Function  Tag=dotview  FunctionName=ltpdasim
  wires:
  dotview/1 -> Terminator/1
  In1/1 -> dotview/1

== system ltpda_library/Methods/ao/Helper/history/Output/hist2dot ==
  In1 : Inport  OutDataType=sfix(16)  OutScaling=2^0
  Terminator : Terminator
  hist2dot : M-S-Function  Tag=hist2dot  FunctionName=ltpdasim
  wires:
  hist2dot/1 -> Terminator/1
  In1/1 -> hist2dot/1

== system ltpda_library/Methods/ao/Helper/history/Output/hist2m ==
  In1 : Inport  OutDataType=sfix(16)  OutScaling=2^0
  Terminator : Terminator
  hist2m : M-S-Function  Tag=hist2m  FunctionName=ltpdasim
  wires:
  hist2m/1 -> Terminator/1
  In1/1 -> hist2m/1

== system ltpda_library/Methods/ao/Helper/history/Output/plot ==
  In1 : Inport  OutDataType=sfix(16)  OutScaling=2^0
  Terminator : Terminator
  plot : M-S-Function  Tag=plot  FunctionName=ltpdasim
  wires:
  plot/1 -> Terminator/1
  In1/1 -> plot/1

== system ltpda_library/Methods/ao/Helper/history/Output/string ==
  In1 : Inport  OutDataType=sfix(16)  OutScaling=2^0
  Terminator : Terminator
  string : M-S-Function  Tag=string  FunctionName=ltpdasim
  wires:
  string/1 -> Terminator/1
  In1/1 -> string/1

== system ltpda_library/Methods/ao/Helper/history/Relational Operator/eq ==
  In1 : Inport  OutDataType=sfix(16)  OutScaling=2^0
  eq : M-S-Function  Tag=eq  FunctionName=ltpdasim
  Out1 : Outport  OutDataType=sfix(16)  OutScaling=2^0
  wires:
  In1/1 -> eq/1
  eq/1 -> Out1/1

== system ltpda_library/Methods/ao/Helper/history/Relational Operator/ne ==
  In1 : Inport  OutDataType=sfix(16)  OutScaling=2^0
  ne : M-S-Function  Tag=ne  FunctionName=ltpdasim
  Out1 : Outport  OutDataType=sfix(16)  OutScaling=2^0
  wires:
  In1/1 -> ne/1
  ne/1 -> Out1/1

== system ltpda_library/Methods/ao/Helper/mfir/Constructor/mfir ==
  Ground : Ground
  mfir : M-S-Function  Tag=mfir  FunctionName=ltpdasim
  Out1 : Outport  OutDataType=sfix(16)  OutScaling=2^0
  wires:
  Ground/1 -> mfir/1
  mfir/1 -> Out1/1

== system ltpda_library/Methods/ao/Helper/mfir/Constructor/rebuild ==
  Ground : Ground
  rebuild : M-S-Function  Tag=rebuild  FunctionName=ltpdasim
  Out1 : Outport  OutDataType=sfix(16)  OutScaling=2^0
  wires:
  Ground/1 -> rebuild/1
  rebuild/1 -> Out1/1

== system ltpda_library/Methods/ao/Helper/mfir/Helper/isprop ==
  In1 : Inport  OutDataType=sfix(16)  OutScaling=2^0
  isprop : M-S-Function  Tag=isprop  FunctionName=ltpdasim
  Out1 : Outport  OutDataType=sfix(16)  OutScaling=2^0
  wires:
  In1/1 -> isprop/1
  isprop/1 -> Out1/1

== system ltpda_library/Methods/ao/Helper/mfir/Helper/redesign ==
  In1 : Inport  OutDataType=sfix(16)  OutScaling=2^0
  redesign : M-S-Function  Tag=redesign  FunctionName=ltpdasim
  Out1 : Outport  OutDataType=sfix(16)  OutScaling=2^0
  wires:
  In1/1 -> redesign/1
  redesign/1 -> Out1/1

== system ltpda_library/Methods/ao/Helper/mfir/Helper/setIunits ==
  In1 : Inport  OutDataType=sfix(16)  OutScaling=2^0
  setIunits : M-S-Function  Tag=setIunits  FunctionName=ltpdasim
  Out1 : Outport  OutDataType=sfix(16)  OutScaling=2^0
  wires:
  In1/1 -> setIunits/1
  setIunits/1 -> Out1/1

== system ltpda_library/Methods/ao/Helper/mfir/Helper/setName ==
  In1 : Inport  OutDataType=sfix(16)  OutScaling=2^0
  setName : M-S-Function  Tag=setName  FunctionName=ltpdasim
  Out1 : Outport  OutDataType=sfix(16)  OutScaling=2^0
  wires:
  In1/1 -> setName/1
  setName/1 -> Out1/1

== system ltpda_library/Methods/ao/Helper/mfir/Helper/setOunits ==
  In1 : Inport  OutDataType=sfix(16)  OutScaling=2^0
  setOunits : M-S-Function  Tag=setOunits  FunctionName=ltpdasim
  Out1 : Outport  OutDataType=sfix(16)  OutScaling=2^0
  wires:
  In1/1 -> setOunits/1
  setOunits/1 -> Out1/1

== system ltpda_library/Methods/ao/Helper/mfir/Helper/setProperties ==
  In1 : Inport  OutDataType=sfix(16)  OutScaling=2^0
  setProperties : M-S-Function  Tag=setProperties  FunctionName=ltpdasim
  Out1 : Outport  OutDataType=sfix(16)  OutScaling=2^0
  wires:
  In1/1 -> setProperties/1
  setProperties/1 -> Out1/1

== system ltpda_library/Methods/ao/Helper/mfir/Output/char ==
  In1 : Inport  OutDataType=sfix(16)  OutScaling=2^0
  Terminator : Terminator
  char : M-S-Function  Tag=char  FunctionName=ltpdasim
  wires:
  char/1 -> Terminator/1
  In1/1 -> char/1

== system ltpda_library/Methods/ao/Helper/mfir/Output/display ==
  In1 : Inport  OutDataType=sfix(16)  OutScaling=2^0
  Terminator : Terminator
  display : M-S-Function  Tag=display  FunctionName=ltpdasim
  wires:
  display/1 -> Terminator/1
  In1/1 -> display/1

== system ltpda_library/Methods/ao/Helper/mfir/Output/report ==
  In1 : Inport  OutDataType=sfix(16)  OutScaling=2^0
  Terminator : Terminator
  report : M-S-Function  Tag=report  FunctionName=ltpdasim
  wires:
  report/1 -> Terminator/1
  In1/1 -> report/1

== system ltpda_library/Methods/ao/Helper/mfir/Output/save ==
  In1 : Inport  OutDataType=sfix(16)  OutScaling=2^0
  Terminator : Terminator
  save : M-S-Function  Tag=save  FunctionName=ltpdasim
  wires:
  save/1 -> Terminator/1
  In1/1 -> save/1

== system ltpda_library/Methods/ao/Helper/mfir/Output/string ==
  In1 : Inport  OutDataType=sfix(16)  OutScaling=2^0
  Terminator : Terminator
  string : M-S-Function  Tag=string  FunctionName=ltpdasim
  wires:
  string/1 -> Terminator/1
  In1/1 -> string/1

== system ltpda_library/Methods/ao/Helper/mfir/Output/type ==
  In1 : Inport  OutDataType=sfix(16)  OutScaling=2^0
  Terminator : Terminator
  type : M-S-Function  Tag=type  FunctionName=ltpdasim
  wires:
  type/1 -> Terminator/1
  In1/1 -> type/1

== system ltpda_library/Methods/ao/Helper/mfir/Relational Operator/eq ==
  In1 : Inport  OutDataType=sfix(16)  OutScaling=2^0
  eq : M-S-Function  Tag=eq  FunctionName=ltpdasim
  Out1 : Outport  OutDataType=sfix(16)  OutScaling=2^0
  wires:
  In1/1 -> eq/1
  eq/1 -> Out1/1

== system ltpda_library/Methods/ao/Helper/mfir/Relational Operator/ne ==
  In1 : Inport  OutDataType=sfix(16)  OutScaling=2^0
  ne : M-S-Function  Tag=ne  FunctionName=ltpdasim
  Out1 : Outport  OutDataType=sfix(16)  OutScaling=2^0
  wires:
  In1/1 -> ne/1
  ne/1 -> Out1/1

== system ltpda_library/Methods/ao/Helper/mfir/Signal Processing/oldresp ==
  In1 : Inport  OutDataType=sfix(16)  OutScaling=2^0
  oldresp : M-S-Function  Tag=oldresp  FunctionName=ltpdasim
  Out1 : Outport  OutDataType=sfix(16)  OutScaling=2^0
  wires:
  In1/1 -> oldresp/1
  oldresp/1 -> Out1/1

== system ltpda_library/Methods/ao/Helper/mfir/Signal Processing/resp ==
  In1 : Inport  OutDataType=sfix(16)  OutScaling=2^0
  resp : M-S-Function  Tag=resp  FunctionName=ltpdasim
  Out1 : Outport  OutDataType=sfix(16)  OutScaling=2^0
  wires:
  In1/1 -> resp/1
  resp/1 -> Out1/1

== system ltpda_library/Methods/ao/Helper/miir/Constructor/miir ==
  Ground : Ground
  miir : M-S-Function  Tag=miir  FunctionName=ltpdasim
  Out1 : Outport  OutDataType=sfix(16)  OutScaling=2^0
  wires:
  Ground/1 -> miir/1
  miir/1 -> Out1/1

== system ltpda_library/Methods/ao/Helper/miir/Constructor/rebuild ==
  Ground : Ground
  rebuild : M-S-Function  Tag=rebuild  FunctionName=ltpdasim
  Out1 : Outport  OutDataType=sfix(16)  OutScaling=2^0
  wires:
  Ground/1 -> rebuild/1
  rebuild/1 -> Out1/1

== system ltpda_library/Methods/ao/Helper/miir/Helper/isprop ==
  In1 : Inport  OutDataType=sfix(16)  OutScaling=2^0
  isprop : M-S-Function  Tag=isprop  FunctionName=ltpdasim
  Out1 : Outport  OutDataType=sfix(16)  OutScaling=2^0
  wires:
  In1/1 -> isprop/1
  isprop/1 -> Out1/1

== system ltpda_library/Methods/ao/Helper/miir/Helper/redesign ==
  In1 : Inport  OutDataType=sfix(16)  OutScaling=2^0
  redesign : M-S-Function  Tag=redesign  FunctionName=ltpdasim
  Out1 : Outport  OutDataType=sfix(16)  OutScaling=2^0
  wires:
  In1/1 -> redesign/1
  redesign/1 -> Out1/1

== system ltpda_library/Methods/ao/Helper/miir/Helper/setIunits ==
  In1 : Inport  OutDataType=sfix(16)  OutScaling=2^0
  setIunits : M-S-Function  Tag=setIunits  FunctionName=ltpdasim
  Out1 : Outport  OutDataType=sfix(16)  OutScaling=2^0
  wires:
  In1/1 -> setIunits/1
  setIunits/1 -> Out1/1

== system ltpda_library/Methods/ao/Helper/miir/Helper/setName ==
  In1 : Inport  OutDataType=sfix(16)  OutScaling=2^0
  setName : M-S-Function  Tag=setName  FunctionName=ltpdasim
  Out1 : Outport  OutDataType=sfix(16)  OutScaling=2^0
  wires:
  In1/1 -> setName/1
  setName/1 -> Out1/1

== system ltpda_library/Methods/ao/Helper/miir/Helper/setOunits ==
  In1 : Inport  OutDataType=sfix(16)  OutScaling=2^0
  setOunits : M-S-Function  Tag=setOunits  FunctionName=ltpdasim
  Out1 : Outport  OutDataType=sfix(16)  OutScaling=2^0
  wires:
  In1/1 -> setOunits/1
  setOunits/1 -> Out1/1

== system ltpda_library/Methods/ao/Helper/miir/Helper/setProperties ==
  In1 : Inport  OutDataType=sfix(16)  OutScaling=2^0
  setProperties : M-S-Function  Tag=setProperties  FunctionName=ltpdasim
  Out1 : Outport  OutDataType=sfix(16)  OutScaling=2^0
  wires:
  In1/1 -> setProperties/1
  setProperties/1 -> Out1/1

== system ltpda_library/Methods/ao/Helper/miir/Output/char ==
  In1 : Inport  OutDataType=sfix(16)  OutScaling=2^0
  Terminator : Terminator
  char : M-S-Function  Tag=char  FunctionName=ltpdasim
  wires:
  char/1 -> Terminator/1
  In1/1 -> char/1

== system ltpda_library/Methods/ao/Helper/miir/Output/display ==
  In1 : Inport  OutDataType=sfix(16)  OutScaling=2^0
  Terminator : Terminator
  display : M-S-Function  Tag=display  FunctionName=ltpdasim
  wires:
  display/1 -> Terminator/1
  In1/1 -> display/1

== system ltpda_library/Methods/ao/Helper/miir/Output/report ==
  In1 : Inport  OutDataType=sfix(16)  OutScaling=2^0
  Terminator : Terminator
  report : M-S-Function  Tag=report  FunctionName=ltpdasim
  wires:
  report/1 -> Terminator/1
  In1/1 -> report/1

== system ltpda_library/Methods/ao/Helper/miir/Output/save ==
  In1 : Inport  OutDataType=sfix(16)  OutScaling=2^0
  Terminator : Terminator
  save : M-S-Function  Tag=save  FunctionName=ltpdasim
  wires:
  save/1 -> Terminator/1
  In1/1 -> save/1

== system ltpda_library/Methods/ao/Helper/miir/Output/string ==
  In1 : Inport  OutDataType=sfix(16)  OutScaling=2^0
  Terminator : Terminator
  string : M-S-Function  Tag=string  FunctionName=ltpdasim
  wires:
  string/1 -> Terminator/1
  In1/1 -> string/1

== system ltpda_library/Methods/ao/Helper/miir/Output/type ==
  In1 : Inport  OutDataType=sfix(16)  OutScaling=2^0
  Terminator : Terminator
  type : M-S-Function  Tag=type  FunctionName=ltpdasim
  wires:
  type/1 -> Terminator/1
  In1/1 -> type/1

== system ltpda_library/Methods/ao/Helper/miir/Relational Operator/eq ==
  In1 : Inport  OutDataType=sfix(16)  OutScaling=2^0
  eq : M-S-Function  Tag=eq  FunctionName=ltpdasim
  Out1 : Outport  OutDataType=sfix(16)  OutScaling=2^0
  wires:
  In1/1 -> eq/1
  eq/1 -> Out1/1

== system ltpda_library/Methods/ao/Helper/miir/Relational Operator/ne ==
  In1 : Inport  OutDataType=sfix(16)  OutScaling=2^0
  ne : M-S-Function  Tag=ne  FunctionName=ltpdasim
  Out1 : Outport  OutDataType=sfix(16)  OutScaling=2^0
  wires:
  In1/1 -> ne/1
  ne/1 -> Out1/1

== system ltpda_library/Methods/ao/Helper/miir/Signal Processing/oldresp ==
  In1 : Inport  OutDataType=sfix(16)  OutScaling=2^0
  oldresp : M-S-Function  Tag=oldresp  FunctionName=ltpdasim
  Out1 : Outport  OutDataType=sfix(16)  OutScaling=2^0
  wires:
  In1/1 -> oldresp/1
  oldresp/1 -> Out1/1

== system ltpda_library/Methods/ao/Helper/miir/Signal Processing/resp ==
  In1 : Inport  OutDataType=sfix(16)  OutScaling=2^0
  resp : M-S-Function  Tag=resp  FunctionName=ltpdasim
  Out1 : Outport  OutDataType=sfix(16)  OutScaling=2^0
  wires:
  In1/1 -> resp/1
  resp/1 -> Out1/1

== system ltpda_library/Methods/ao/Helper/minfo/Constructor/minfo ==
  Ground : Ground
  minfo : M-S-Function  Tag=minfo  FunctionName=ltpdasim
  Out1 : Outport  OutDataType=sfix(16)  OutScaling=2^0
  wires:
  Ground/1 -> minfo/1
  minfo/1 -> Out1/1

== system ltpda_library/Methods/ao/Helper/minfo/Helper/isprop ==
  In1 : Inport  OutDataType=sfix(16)  OutScaling=2^0
  isprop : M-S-Function  Tag=isprop  FunctionName=ltpdasim
  Out1 : Outport  OutDataType=sfix(16)  OutScaling=2^0
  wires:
  In1/1 -> isprop/1
  isprop/1 -> Out1/1

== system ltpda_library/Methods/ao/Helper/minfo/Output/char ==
  In1 : Inport  OutDataType=sfix(16)  OutScaling=2^0
  Terminator : Terminator
  char : M-S-Function  Tag=char  FunctionName=ltpdasim
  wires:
  char/1 -> Terminator/1
  In1/1 -> char/1

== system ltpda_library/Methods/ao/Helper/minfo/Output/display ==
  In1 : Inport  OutDataType=sfix(16)  OutScaling=2^0
  Terminator : Terminator
  display : M-S-Function  Tag=display  FunctionName=ltpdasim
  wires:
  display/1 -> Terminator/1
  In1/1 -> display/1

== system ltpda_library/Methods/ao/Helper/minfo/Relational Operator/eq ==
  In1 : Inport  OutDataType=sfix(16)  OutScaling=2^0
  eq : M-S-Function  Tag=eq  FunctionName=ltpdasim
  Out1 : Outport  OutDataType=sfix(16)  OutScaling=2^0
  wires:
  In1/1 -> eq/1
  eq/1 -> Out1/1

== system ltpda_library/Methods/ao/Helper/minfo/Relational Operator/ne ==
  In1 : Inport  OutDataType=sfix(16)  OutScaling=2^0
  ne : M-S-Function  Tag=ne  FunctionName=ltpdasim
  Out1 : Outport  OutDataType=sfix(16)  OutScaling=2^0
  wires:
  In1/1 -> ne/1
  ne/1 -> Out1/1

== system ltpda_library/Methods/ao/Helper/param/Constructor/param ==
  Ground : Ground
  param : M-S-Function  Tag=param  FunctionName=ltpdasim
  Out1 : Outport  OutDataType=sfix(16)  OutScaling=2^0
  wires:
  Ground/1 -> param/1
  param/1 -> Out1/1

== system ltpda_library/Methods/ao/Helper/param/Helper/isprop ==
  In1 : Inport  OutDataType=sfix(16)  OutScaling=2^0
  isprop : M-S-Function  Tag=isprop  FunctionName=ltpdasim
  Out1 : Outport  OutDataType=sfix(16)  OutScaling=2^0
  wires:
  In1/1 -> isprop/1
  isprop/1 -> Out1/1

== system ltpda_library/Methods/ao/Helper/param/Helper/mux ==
  In1 : Inport  OutDataType=sfix(16)  OutScaling=2^0
  mux : M-S-Function  Tag=mux  FunctionName=ltpdasim
  Out1 : Outport  OutDataType=sfix(16)  OutScaling=2^0
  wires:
  In1/1 -> mux/1
  mux/1 -> Out1/1

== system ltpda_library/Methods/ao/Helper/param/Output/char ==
  In1 : Inport  OutDataType=sfix(16)  OutScaling=2^0
  Terminator : Terminator
  char : M-S-Function  Tag=char  FunctionName=ltpdasim
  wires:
  char/1 -> Terminator/1
  In1/1 -> char/1

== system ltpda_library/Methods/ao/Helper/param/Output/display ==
  In1 : Inport  OutDataType=sfix(16)  OutScaling=2^0
  Terminator : Terminator
  display : M-S-Function  Tag=display  FunctionName=ltpdasim
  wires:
  display/1 -> Terminator/1
  In1/1 -> display/1

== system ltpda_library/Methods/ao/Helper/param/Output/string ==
  In1 : Inport  OutDataType=sfix(16)  OutScaling=2^0
  Terminator : Terminator
  string : M-S-Function  Tag=string  FunctionName=ltpdasim
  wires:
  string/1 -> Terminator/1
  In1/1 -> string/1

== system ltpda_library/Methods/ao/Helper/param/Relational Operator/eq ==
  In1 : Inport  OutDataType=sfix(16)  OutScaling=2^0
  eq : M-S-Function  Tag=eq  FunctionName=ltpdasim
  Out1 : Outport  OutDataType=sfix(16)  OutScaling=2^0
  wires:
  In1/1 -> eq/1
  eq/1 -> Out1/1
